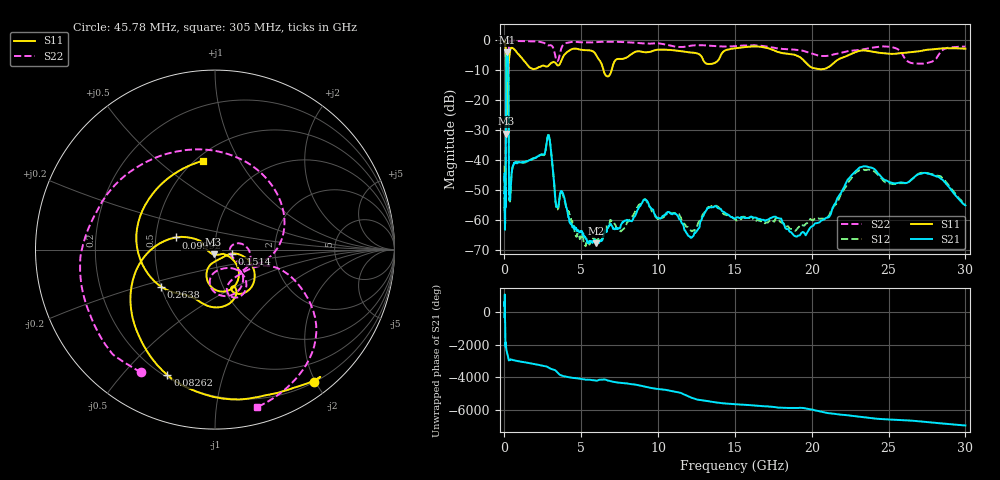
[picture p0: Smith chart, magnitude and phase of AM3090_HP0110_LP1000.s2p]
! Date/Time: Thu, Feb 28, 2019 2:00 PM
! Network Analyzer: Agilent Technologies E8364B Rev: A.07.50.67
! Sweep from 0.010 to 30.000 GHz, 1601 Points, Sweep Type: LOG
! Power Supply: 5.023 V, 0.002 A
# Hz S DB R 50
!freq MagS11 AngS11 MagS21 AngS21 MagS12 AngS12 MagS22 AngS22
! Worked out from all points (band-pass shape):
!   1601 points, 10 MHz to 30 GHz, reference 50 ohm
!   highest |S21| = -4.12 dB at 156 MHz (marker M1); lowest = -67.6 dB at 5.989 GHz (marker M2)
!   |S21| within 3 dB of the highest: 110.9 MHz to 240.1 MHz (129.2 MHz wide, 73.6 % of centre)
!   lowest |S11| = -31.1 dB at 107.7 MHz (marker M3), VSWR 1.06, Z = 49.1 - j2.63 ohm
!   |S11| at or under -10 dB: 98.35 MHz to 224.2 MHz (125.9 MHz wide, 78 % of centre); 233.7 MHz to 255.9 MHz (22.19 MHz wide, 9.06 % of centre); 6.447 GHz to 6.977 GHz (529.9 MHz wide, 7.89 % of centre)
!   |S22| runs from -21.7 to -0.1 dB; largest |S21 - S12| = 0.012
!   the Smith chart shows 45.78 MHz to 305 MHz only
!   S11 on the Smith chart (normalised r, x): 45.78 MHz: 0.21, -1.98; 82.62 MHz: 0.21, -0.67; 99.92 MHz: 0.64, +0.09; 151.4 MHz: 1.21, -0.05; 263.8 MHz: 0.50, -0.24; 305 MHz: 0.54, +0.72
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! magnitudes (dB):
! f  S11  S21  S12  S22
! 10 MHz  -0.2  -46.8  -41.7  -0.7
! 38.04 MHz  -0.5  -57.8  -58.9  -1.4
! 45.78 MHz  -0.7  -54.5  -50.1  -2.0
! 82.62 MHz  -2.5  -51.7  -49.8  -4.8
! 99.92 MHz  -12.8  -16.1  -16.1  -11.3
! 107.7 MHz  -31.1  -8.3  -8.3  -21.2
! 123.3 MHz  -12.5  -5.4  -5.3  -14.8
! 144.7 MHz  -24.7  -4.3  -4.3  -15.3
! 151.4 MHz  -20.3  -4.2  -4.1  -15.1
! 156 MHz  -15.7  -4.1  -4.1  -14.3
! 236.3 MHz  -10.2  -6.7  -6.7  -11.3
! 263.8 MHz  -8.8  -17.8  -17.8  -8.0
! 305 MHz  -6.0  -50.6  -51.3  -0.8
! 550.5 MHz  -2.7  -41.9  -41.8  -0.2
! 2.084 GHz  -9.5  -39.0  -39.0  -0.5
! 2.884 GHz  -8.4  -31.7  -31.7  -1.8
! 3.402 GHz  -8.1  -55.6  -56.5  -6.9
! 5.989 GHz  -5.2  -67.6  -66.8  -0.7
! 7.926 GHz  -5.9  -60.0  -61.5  -0.7
! 19.31 GHz  -6.0  -64.2  -62.1  -3.4
! 23.48 GHz  -3.5  -42.0  -43.3  -3.0
! 30 GHz  -2.9  -55.0  -54.9  -2.2
